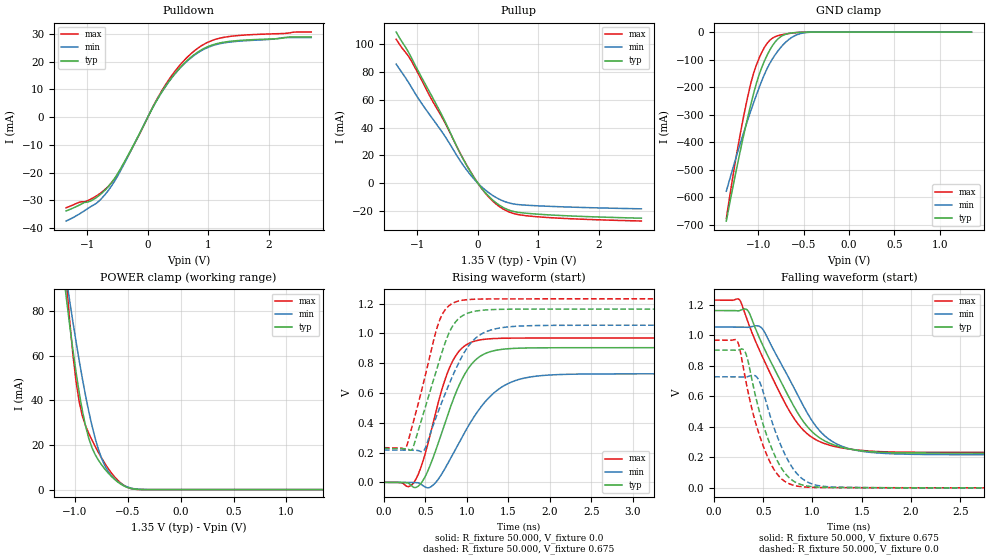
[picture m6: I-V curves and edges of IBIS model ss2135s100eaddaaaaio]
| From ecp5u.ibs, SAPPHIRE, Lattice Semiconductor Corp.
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|   Model ss2135s100eaddaaaaio
| Clamp models does not include dynamic input termination. Please
| use correspodent INPUT models to simulate input termination.
[Model] ss2135s100eaddaaaaio
Model_type I/O
Polarity   Non-Inverting
Enable   Active-Low
Vinl =  0.575V
Vinh =  0.775V
Vmeas =  0.675V
Cref =  30.000pF
Rref =  50.000
Vref =  0.675V
C_comp   5.000pF   4.000pF   5.500pF
[Temperature Range]   25.000   0.125k   -40.000
[Voltage Range]   1.350V   1.280V   1.420V
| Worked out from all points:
|   slope of the pulldown table from 0 to 0.203 V, typ, clamps not added: 25.1 ohm
|   slope of the pullup table from 0 to 0.203 V, typ, clamps not added: 19.5 ohm
|   GND clamp passes 1 mA (typ) near -0.54 V on its own axis
|   POWER clamp passes 1 mA (typ) near -0.51 V on its own axis
|   rising waveform, R_fixture 50.000, V_fixture 0.0: 20-80 % time 368ps typ, 503ps min, 297ps max; typ from 0 V to 0.904 V
|   rising waveform, R_fixture 50.000, V_fixture 0.675: 20-80 % time 314ps typ, 391ps min, 269ps max; typ from 0.227 V to 1.16 V
|   falling waveform, R_fixture 50.000, V_fixture 0.675: 20-80 % time 465ps typ, 440ps min, 461ps max; typ from 1.16 V to 0.227 V
|   falling waveform, R_fixture 50.000, V_fixture 0.0: 20-80 % time 259ps typ, 262ps min, 250ps max; typ from 0.904 V to 0 V
[Pulldown]
|Voltage   I(typ)   I(min)   I(max)
-1.35V    -33.78mA   -37.41mA   -32.64mA
-850mV    -28.97mA   -31.05mA   -28.4mA
-600mV    -23.63mA   -24.79mA   -23.65mA
-350mV    -14.66mA   -15.1mA    -14.92mA
50mV      2.157mA    2.138mA    2.25mA
200mV     7.987mA    7.913mA    8.357mA
450mV     15.76mA    15.6mA     16.57mA
750mV     22.25mA    22mA       23.54mA
1V        25.47mA    25.19mA    27.06mA
1.3V      27.15mA    26.89mA    28.91mA
2.25V     28.55mA    28.68mA    30.15mA
2.7V      28.9mA     28.68mA    30.66mA
[Pullup]
|Voltage   I(typ)   I(min)   I(max)
-1.35V    108.6mA    85.56mA    103.4mA
-1.1V     90.26mA    69.04mA    87.95mA
-800mV    65.64mA    49.36mA    62.97mA
-600mV    49.28mA    37.29mA    47.89mA
-300mV    22.03mA    16.59mA    22.16mA
-150mV    10.08mA    7.445mA    10.4mA
100mV     -5.613mA   -4.06mA    -5.96mA
300mV     -14.08mA   -10.26mA   -14.96mA
550mV     -19.83mA   -14.55mA   -21.23mA
800mV     -21.55mA   -15.77mA   -23.33mA
1.5V      -23.43mA   -17.1mA    -25.43mA
2.7V      -25.1mA    -18.37mA   -27.13mA
[GND_clamp]
|Voltage   I(typ)   I(min)   I(max)
-1.35V    -687.3mA   -578.9mA   -678.1mA
-1.26V    -534.3mA   -475.1mA   -489.7mA
-1.2V     -438.1mA   -409.1mA   -376.7mA
-1.08V    -262.9mA   -286.2mA   -185.9mA
-1.02V    -187.7mA   -229.9mA   -120.7mA
-960mV    -129.1mA   -177.6mA   -73.95mA
-900mV    -83.6mA    -132.1mA   -40.76mA
-840mV    -48.57mA   -96.56mA   -21.66mA
-750mV    -16.65mA   -55.68mA   -10.64mA
-660mV    -4.958mA   -26.68mA   -5.448mA
-480mV    -317.7uA   -2.229mA   -341.9uA
1.35V     0A         0A         0A
[POWER_clamp]
|Voltage   I(typ)   I(min)   I(max)
-1.35V    211.5mA    193mA      324.9mA
-1.08V    85.33mA    94.25mA    92.93mA
-1.05V    73.76mA    84.65mA    75.65mA
-990mV    52.73mA    66.45mA    48.6mA
-960mV    43.53mA    57.9mA     39.38mA
-930mV    35.42mA    49.79mA    33mA
-840mV    18.88mA    28.82mA    22.31mA
-750mV    11.24mA    14.22mA    14.3mA
-660mV    6.13mA     6.499mA    7.742mA
-570mV    2.538mA    2.795mA    3.049mA
-390mV    57.41uA    134.8uA    35.81uA
1.35V     0A         0A         0A
[Ramp]
| variable   typ   min   max
dV/dt_r 0.542/0.372n   0.437/0.507n   0.581/0.299n
dV/dt_f 0.511/0.477n   0.485/0.422n   0.546/0.508n
R_load = 50.000
[Rising Waveform]
R_fixture= 50.000
V_fixture= 0.0
V_fixture_min= 0.0
V_fixture_max= 0.0
|time   V(typ)   V(min)   V(max)
0s        0V         0V         0V
306ps     -9.832mV   -698.3uV   -27.3mV
444ps     -8.644mV   -12.22mV   98.03mV
590ps     161.2mV    -19.77mV   392.1mV
809ps     515.8mV    166.6mV    792mV
986ps     737.2mV    347.6mV    920.4mV
1.159ns   845.3mV    498mV      955.8mV
1.51ns    897mV      666.4mV    967.7mV
2.056ns   903.2mV    722mV      968.6mV
10ns      903.5mV    728.2mV    968.6mV
[Rising Waveform]
R_fixture= 50.000
V_fixture= 0.675
V_fixture_min= 0.642
V_fixture_max= 0.710
|time   V(typ)   V(min)   V(max)
0s        227.4mV    216.8mV    232.4mV
254ps     225.8mV    216.7mV    222.6mV
347ps     227.6mV    215.7mV    389.8mV
487ps     482mV      217.4mV    690.2mV
672ps     823.6mV    500.8mV    1.089V
804ps     1.025V     683mV      1.194V
934ps     1.113V     837mV      1.221V
1.192ns   1.155V     1V         1.23V
1.659ns   1.162V     1.049V     1.231V
10ns      1.163V     1.054V     1.231V
[Falling Waveform]
R_fixture= 50.000
V_fixture= 0.675
V_fixture_min= 0.642
V_fixture_max= 0.710
|time   V(typ)   V(min)   V(max)
0s        1.163V     1.054V     1.231V
257ps     1.162V     1.055V     1.234V
347ps     1.159V     1.053V     1.082V
484ps     949.4mV    1.048V     869.9mV
728ps     634.7mV    758.8mV    547.5mV
888ps     452.5mV    560.9mV    391.4mV
1.087ns   321.7mV    364.6mV    299.2mV
1.328ns   261.2mV    265.8mV    258.8mV
2.209ns   227.9mV    218.3mV    232.6mV
10ns      227.4mV    216.8mV    232.4mV
[Falling Waveform]
R_fixture= 50.000
V_fixture= 0.0
V_fixture_min= 0.0
V_fixture_max= 0.0
|time   V(typ)   V(min)   V(max)
0s        903.5mV    728.2mV    968.6mV
239ps     903.1mV    728.2mV    958.5mV
327ps     873.2mV    727.5mV    686.1mV
435ps     564.4mV    725.7mV    398.6mV
529ps     355.1mV    562.5mV    225.8mV
640ps     180.7mV    339.5mV    91.38mV
859ps     27.17mV    81.38mV    9.9mV
1.047ns   5.169mV    16.42mV    2.349mV
1.427ns   1.494mV    2.294mV    1.124mV
10ns      0V         0V         0V
